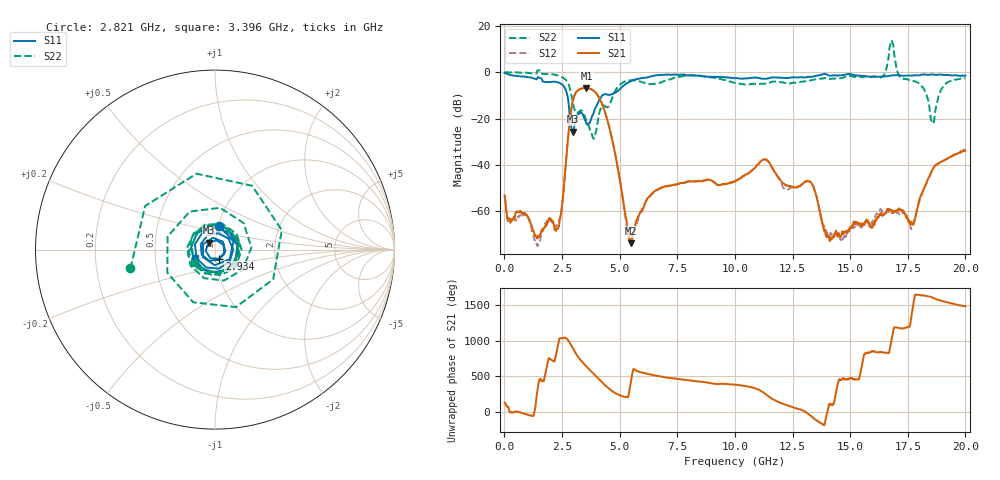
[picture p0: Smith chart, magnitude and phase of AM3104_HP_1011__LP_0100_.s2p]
!Created with skrf (http://scikit-rf.org).
# Hz S RI R 50.0
!freq ReS11 ImS11 ReS21 ImS21 ReS12 ImS12 ReS22 ImS22
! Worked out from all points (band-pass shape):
!   1601 points, 10 MHz to 20 GHz, reference 50 ohm
!   highest |S21| = -6.79 dB at 3.558 GHz (marker M1); lowest = -73.8 dB at 5.495 GHz (marker M2)
!   |S21| within 3 dB of the highest: 3.052 GHz to 4.035 GHz (982.9 MHz wide, 27.7 % of centre)
!   lowest |S11| = -25.7 dB at 2.971 GHz (marker M3), VSWR 1.11, Z = 46.4 + j3.51 ohm
!   |S11| at or under -10 dB: 2.733 GHz to 4.251 GHz (1.518 GHz wide, 43.5 % of centre)
!   |S22| runs from -28.7 to 13.6 dB; largest |S21 - S12| = 0.019
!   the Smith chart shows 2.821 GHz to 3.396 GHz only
!   S11 on the Smith chart (normalised r, x): 2.821 GHz: 1.01, +0.27; 2.934 GHz: 1.04, -0.11; 3.396 GHz: 0.79, -0.08
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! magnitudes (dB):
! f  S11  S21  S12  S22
! 10 MHz  -0.3  -53.2  -53.2  0.0
! 1.434 GHz  -2.5  -71.0  -74.9  0.7
! 2.284 GHz  -4.3  -67.3  -66.1  -1.3
! 2.821 GHz  -17.4  -22.3  -22.4  -6.3
! 2.934 GHz  -25.0  -14.1  -14.2  -11.2
! 2.971 GHz  -25.7  -12.3  -12.3  -13.3
! 3.346 GHz  -17.6  -7.0  -7.1  -16.5
! 3.396 GHz  -18.1  -6.9  -7.0  -17.0
! 3.558 GHz  -22.0  -6.8  -6.9  -21.1
! 3.883 GHz  -17.3  -8.1  -8.1  -28.7
! 4.42 GHz  -9.6  -18.9  -19.0  -15.0
! 5.495 GHz  -3.8  -73.8  -72.5  -3.6
! 6.682 GHz  -1.2  -50.5  -50.4  -4.8
! 10.01 GHz  -2.7  -47.1  -47.1  -4.6
! 11.3 GHz  -2.9  -37.5  -37.8  -5.0
! 13.34 GHz  -2.1  -48.1  -48.3  -3.5
! 14.13 GHz  -1.6  -72.8  -70.1  -2.9
! 16.68 GHz  -1.6  -59.2  -60.4  7.2
! 17.71 GHz  -1.5  -65.3  -66.7  -3.8
! 18.58 GHz  -0.9  -41.9  -42.1  -21.8
! 19.05 GHz  -1.1  -38.1  -38.1  -6.0
! 20 GHz  -1.4  -33.9  -33.1  -2.5
